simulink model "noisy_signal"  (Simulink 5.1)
settings: Solver=ode45  StartTime=0.0  StopTime=tmax  RelTol=1e-3
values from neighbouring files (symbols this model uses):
  ampnoise = 0.5    [aliasing.m]    (also in aliasing_w_filter.m; frequency_spectra.m)
  ampsig = 1    [aliasing.m]    (also in aliasing_w_filter.m; frequency_spectra.m)
  Deltat = .001    (= 0.001)    [aliasing.m]    (also in aliasing_w_filter.m; frequency_spectra.m)
  fnoise = 8    [aliasing.m]    (also in aliasing_w_filter.m; frequency_spectra.m)
  fsig = 1    [aliasing.m]    (also in aliasing_w_filter.m; frequency_spectra.m)
  T = .09    (= 0.09)    [aliasing.m]    (also in aliasing_w_filter.m; frequency_spectra.m)

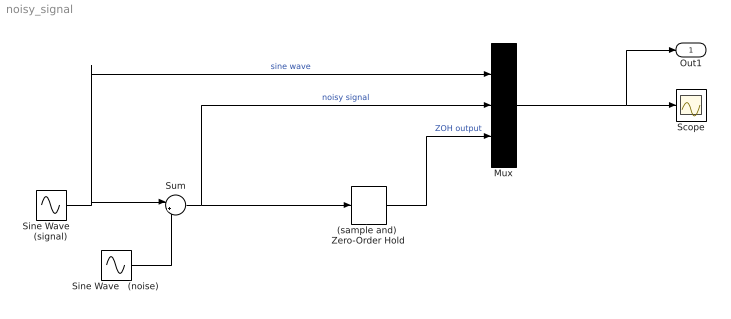
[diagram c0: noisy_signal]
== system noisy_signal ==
  (sample and)  Zero-Order Hold : ZeroOrderHold  SampleTime=T
  Mux : Mux  Inputs=3
  Scope : Scope
  Sine Wave   (noise) : Sin  Amplitude=ampnoise  Frequency=2*pi*fnoise  SampleTime=Deltat
  Sine Wave    (signal) : Sin  Amplitude=ampsig  Frequency=2*pi*fsig  SampleTime=Deltat
  Sum : Sum  Inputs=|++
  Out1 : Outport
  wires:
  Sine Wave    (signal)/1 -> Sum/1, Mux/1  "sine wave"
  Sine Wave   (noise)/1 -> Sum/2
  Sum/1 -> Mux/2, (sample and)  Zero-Order Hold/1  "noisy signal"
  Mux/1 -> Scope/1, Out1/1
  (sample and)  Zero-Order Hold/1 -> Mux/3  "ZOH output"
